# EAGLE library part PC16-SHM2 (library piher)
POTENTIOMETER single carbon potentiometer, 16 mm, S3ROH
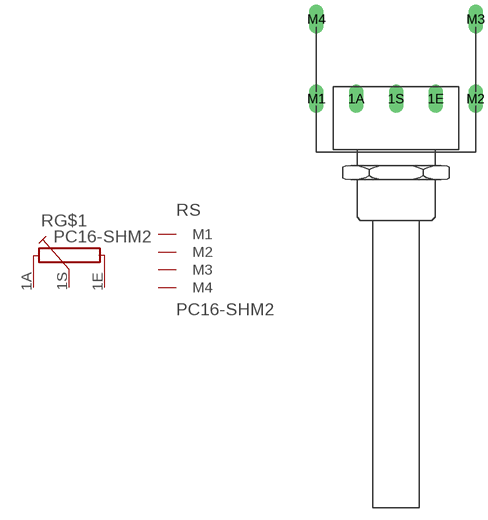
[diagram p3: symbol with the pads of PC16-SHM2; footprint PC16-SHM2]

Designator prefix R; gates G$1=POT S=PC16-M2

## PC16-SHM2 (OC_FARNELL: unknown; OC_NEWARK: unknown)  [PC16-SHM2]
1A  G$1:1A  pas
1E  G$1:1E  pas
1S  G$1:1S  pas
M1  S:M1  pas
M2  S:M2  pas
M3  S:M3  pas
M4  S:M4  pas

## Footprint PC16-SHM2 (pad centres in mm)
POTENTIOMETER single carbon potentiometer, 16 mm
drill 1.2 long: 1A -5,6.5; 1E 5,6.5; 1S 0,6.5; M1 -10,6.5; M2 10,6.5; M3 10,16.5; M4 -10,16.5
